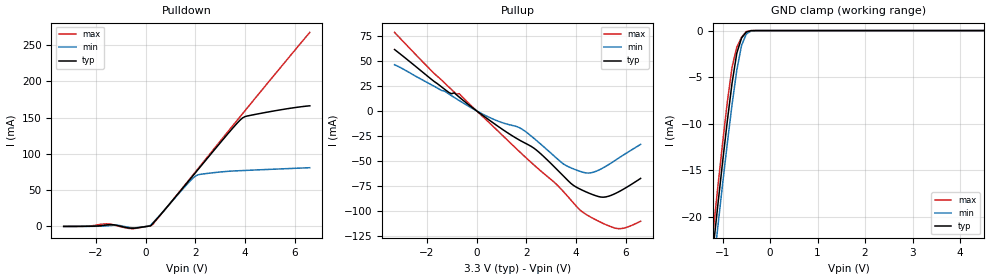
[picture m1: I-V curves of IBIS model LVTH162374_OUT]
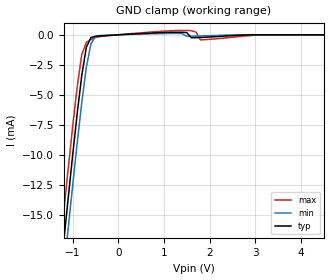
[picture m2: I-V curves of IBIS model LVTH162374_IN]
|   TEXAS INSTRUMENTS INCORPORATED
|   HiRel Division
|   IBIS Model of SN54LVTH162374
|   3.3-V ABT 16-BIT FLIPFLOP WITH 3-STATE OUTPUTS
|   48-pin WD Package
[IBIS Ver]   2.1
[File Name]   lvth162374wd.ibs
[File Rev]   1.0
[Date]   02/8/08
[Source]   File originated at Texas Instruments, Inc.
[Notes]   The following is an IBIS list for the LVTH162374.
|   - This file may be incomplete or may not be fully compliant
|   with the IBIS specification. It will be replaced with a
|   version that is IBIS Revision 3.2 compliant and is complete
|   and accurate.  Please email all questions and comments to
|   sllibis@ti.com.
|   - All test data contained in this file are derived from
|   hspice(tm) simulations.
|   - File created by Ramzi Ammar, SLL Applications.
|   - Disclaimer modified by David Holmgreen, Launch Marketing
|   - WD package parasitics added by Clayton Gibbs, HiRel Applications.
[Disclaimer] Property of Texas Instruments Incorporated.  Unauthorized
   reproduction and/or distribution is strictly prohibited.
   This product is protected under copyright law.
   Created 1999, (C) Copyright 1999, Texas Instruments Inc.,
   All Rights Reserved
   UNLESS THERE IS A SIGNED, WRITTEN AGREEMENT TO THE
   CONTRARY, TEXAS INSTRUMENTS ("TI") IS PROVIDING THE IBIS
   MODELS "AS IS" AND WITHOUT ANY WARRANTY, EXPRESSED OR
   IMPLIED.  TI assumes no liability for:
   1) the accuracy of the IBIS models provided to your
   company;
   2) the proper functioning of these IBIS models in your
   design or for any resulting applications; or
   3) infringement of patents, copyrights or intellectual
   property rights resulting from your use of these IBIS
   models.
   TI provides IBIS Models as a service to our customers.
   You and your company shall not distribute, sell or give
   these models to anyone else without prior written
   permission from TI.
   TI reserves the right to make changes to our products or
   to discontinue any semiconductor product or service
   without notice, and advises our customers to obtain the
   latest version of relevant information to verify, before
   placing orders, that the information being relied on is
   current.
   Please be aware that your receipt and use of the IBIS
   information provided shall serve as acceptance of these
   terms and conditions.  If you do not accept these terms,
   you should return or destroy the IBIS models and any
   other accompanying information immediately.
[Component]   LVTH162374_WD
[Manufacturer]  Texas Instruments, Inc.
[Package]
|   typ   min   max
R_pkg   0.227   0.178   0.322
L_pkg   6.739nH   5.288nH   9.802nH
C_pkg   2.429pF   1.565pF   3.694pF
[Pin]   signal_name   model_name   R_pin   L_pin   C_pin
1   1OE_BAR   NC   0.322   9.802nH   3.217pF
2   1Q1   LVTH162374_OUT   0.311   9.246nH   3.694pF
3   1Q2   LVTH162374_OUT   0.281   8.383nH   3.344pF
4   GND   GND   0.256   7.616nH   2.954pF
5   1Q3   LVTH162374_OUT   0.235   6.904nH   2.400pF
6   1Q4   LVTH162374_OUT   0.216   6.300nH   2.125pF
7   VCC   POWER   0.193   5.587nH   2.147pF
8   1Q5   LVTH162374_OUT   0.188   5.470nH   2.091pF
9   1Q6   LVTH162374_OUT   0.186   5.436nH   1.874pF
10   GND   GND   0.180   5.351nH   1.807pF
11   1Q7   LVTH162374_OUT   0.178   5.288nH   1.929pF
12   1Q8   LVTH162374_OUT   0.180   5.364nH   1.565pF
13   2Q1   LVTH162374_OUT   0.180   5.364nH   1.565pF
14   2Q2   LVTH162374_OUT   0.178   5.288nH   1.929pF
15   GND   GND   0.180   5.351nH   1.807pF
16   2Q3   LVTH162374_OUT   0.186   5.436nH   1.874pF
17   2Q4   LVTH162374_OUT   0.188   5.470nH   2.091pF
18   VCC   POWER   0.193   5.587nH   2.147pF
19   2Q5   LVTH162374_OUT   0.216   6.300nH   2.125pF
20   2Q6   LVTH162374_OUT   0.235   6.904nH   2.400pF
21   GND   GND   0.256   7.616nH   2.954pF
22   2Q7   LVTH162374_OUT   0.281   8.383nH   3.344pF
23   2Q8   LVTH162374_OUT   0.311   9.246nH   3.694pF
24   2OE_BAR   NC   0.322   9.802nH   3.217pF
25   2CLK   NC   0.322   9.802nH   3.217pF
26   2D8   LVTH162374_IN   0.311   9.246nH   3.694pF
27   2D7   LVTH162374_IN   0.281   8.383nH   3.344pF
28   GND   GND   0.256   7.616nH   2.954pF
29   2D6   LVTH162374_IN   0.235   6.904nH   2.400pF
30   2D5   LVTH162374_IN   0.216   6.300nH   2.125pF
31   VCC   POWER   0.193   5.587nH   2.147pF
32   2D4   LVTH162374_IN   0.188   5.470nH   2.091pF
33   2D3   LVTH162374_IN   0.186   5.436nH   1.874pF
34   GND   GND   0.180   5.351nH   1.807pF
35   2D2   LVTH162374_IN   0.178   5.288nH   1.929pF
36   2D1   LVTH162374_IN   0.180   5.364nH   1.565pF
37   1D8   LVTH162374_IN   0.180   5.364nH   1.565pF
38   1D7   LVTH162374_IN   0.178   5.288nH   1.929pF
39   GND   GND   0.180   5.351nH   1.807pF
40   1D6   LVTH162374_IN   0.186   5.436nH   1.874pF
41   1D5   LVTH162374_IN   0.188   5.470nH   2.091pF
42   VCC   POWER   0.193   5.587nH   2.147pF
43   1D4   LVTH162374_IN   0.216   6.300nH   2.125pF
44   1D3   LVTH162374_IN   0.235   6.904nH   2.400pF
45   GND   GND   0.256   7.616nH   2.954pF
46   1D2   LVTH162374_IN   0.281   8.383nH   3.344pF
47   1D1   LVTH162374_IN   0.311   9.246nH   3.694pF
48   1CLK   NC   0.322   9.802nH   3.217pF
| Models and submodels in the file (2): LVTH162374_OUT (3-state), LVTH162374_IN (Input)
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|   Model LVTH162374_OUT
[Model]   LVTH162374_OUT
Model_type   3-state
Polarity   Inverting
Enable   Active-Low
|   typ   min   max
C_comp   9pF   NA   NA
[Voltage range]   3.3   3.0   3.6
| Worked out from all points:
|   slope of the pulldown table from 0 to 0.495 V, typ, clamps not added: 40 ohm
|   slope of the pullup table from 0 to 0.495 V, typ, clamps not added: 55.2 ohm
|   GND clamp passes 1 mA (typ) near -0.61 V on its own axis
| Notes: (1) Vtable = Vcc - Voutput
|   (2) Pullup data includes the effects of the ESD
|   clamping circuitry
[pullup]
|   50C:3.3V:   100C:3V:weak   0C:3.6V:strong
|   Voltage   I(typ)   I(min)   I(max)
-3.3V     61.05mA    45.92mA    78.12mA
-1.7V     29.1mA     24.37mA    37.11mA
-900mV    17.92mA    13.36mA    18.71mA
300mV     -5.464mA   -3.974mA   -6.92mA
1.8V      -30.18mA   -17.84mA   -42.38mA
2.4V      -38.98mA   -29.33mA   -55.96mA
3.5V      -65.09mA   -53.05mA   -80.64mA
4.2V      -78.45mA   -60.6mA    -99.62mA
4.6V      -82.81mA   -61.77mA   -106mA
5.2V      -85.78mA   -55.31mA   -113.4mA
5.8V      -79.61mA   -45.75mA   -117.4mA
6.6V      -67.35mA   -33.43mA   -110mA
[pulldown]
|   50C:3.3V:   100C:3V:weak   0C:3.6V:strong
|   Voltage   I(typ)   I(min)   I(max)
-3.3V     92.7uA     60.9uA     44.3uA
-1.5V     2.392mA    991uA      3.569mA
-1.1V     1.029mA    1.605mA    500.5uA
-700mV    -1.986mA   -1.076mA   -2.56mA
-400mV    -2.134mA   -1.731mA   -2.534mA
100mV     388.4uA    370.5uA    358.3uA
300mV     4.738mA    5.558mA    3.187mA
2V        74.04mA    69.45mA    75.18mA
3.4V      131.5mA    76.18mA    134.5mA
3.9V      149.6mA    77.02mA    155.5mA
5V        158.2mA    78.68mA    201.4mA
6.6V      166.2mA    80.95mA    267.3mA
[gnd clamp]
|   50C:3.3V:   100C:3V:weak   0C:3.6V:strong
|   Voltage   I(typ)   I(min)   I(max)
-3.3V     -167.5mA   -174mA     -161.2mA
-1.2V     -23.52mA   -25.82mA   -21.68mA
-1.1V     -18.76mA   -21.1mA    -16.82mA
-1V       -14.14mA   -16.52mA   -12.12mA
-900mV    -9.713mA   -12.1mA    -7.682mA
-800mV    -5.634mA   -7.938mA   -3.92mA
-700mV    -2.42mA    -4.236mA   -1.774mA
-600mV    -798.4uA   -1.584mA   -716.7uA
-500mV    -157.9uA   -372.6uA   -104.2uA
-400mV    -8.1uA     -38.68uA   -1.238uA
-300mV    -253.1nA   -1.996uA   -31.04nA
6.6V      9.799nA    10.83nA    9.505nA
[ramp]
| variable   typ   min   max
dV/dt_r   9.7744E-01/7.7329E-10  6.7130E-01/1.7654E-09  1.1837E+00/3.1462E-10
dV/dt_f   1.2670E+00/4.7199E-10  1.1366E+00/8.9695E-10  1.3974E+00/2.6900E-10
|   Model LVTH162374_IN
[Model]   LVTH162374_IN
Model_type   Input
Polarity   Inverting
Vinl = 0.8V
Vinh = 2.0V
|   typ   min   max
C_comp   4pF   NA   NA
[Voltage Range]   3.3   3.0   3.6
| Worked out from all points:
|   GND clamp passes 1 mA (typ) near -0.70 V on its own axis
[gnd clamp]
|   50C:3.3V:   100C:3V:weak   0C:3.6V:strong
|   Voltage   I(typ)   I(min)   I(max)
-3.3V     -104.8mA   -107.5mA   -102.3mA
-1.3V     -21.28mA   -23.85mA   -18.78mA
-1.2V     -17.45mA   -20.02mA   -14.97mA
-1.1V     -13.7mA    -16.25mA   -11.25mA
-800mV    -3.378mA   -5.638mA   -1.638mA
-700mV    -1.033mA   -2.696mA   -628.8uA
-600mV    -233.1uA   -754.8uA   -402.2uA
-400mV    -95.77uA   -65.98uA   -147.2uA
600mV     121.7uA    74.16uA    195.2uA
1.6V      -246.5uA   -122uA     340uA
1.8V      -221.7uA   -100.5uA   -421.4uA
6.6V      3.94nA     4.221nA    3.863nA
